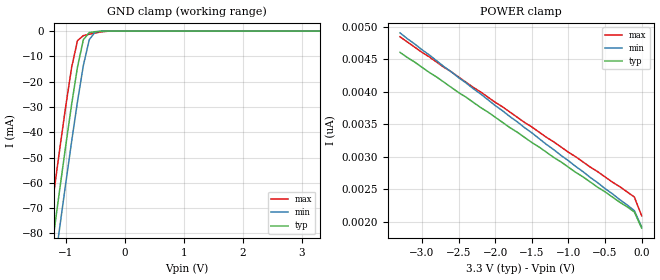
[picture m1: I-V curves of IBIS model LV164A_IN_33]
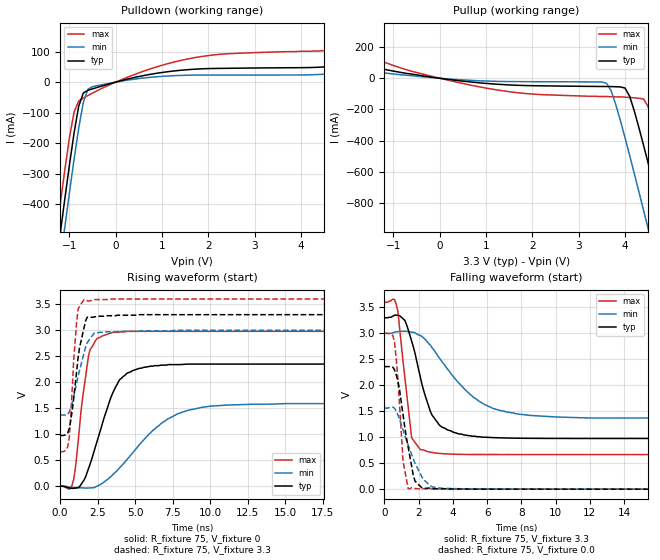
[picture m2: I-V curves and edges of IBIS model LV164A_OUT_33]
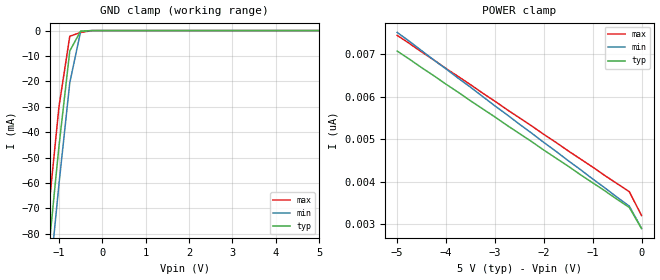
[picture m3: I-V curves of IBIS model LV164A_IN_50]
| TEXAS INSTRUMENTS INCORPORATED
| Standard Linear and Logic Group
| IBIS Model of SN74LV164A
| 8-BIT PARALLEL-OUT SERIAL SHIFT REGISTER
| SOIC 14-pin (D), SOP 14-pin (NS), SSOP 14-pin (DB), TSSOP 14-pin (PW)
| and TVSOP 14-pin (DGV) Package
[IBIS Ver]   3.2
[Comment Char]  |_char
[File Name]   lv164a.ibs
[File Rev]   2.0 H_die
[Date]   May 24, 2000
[Source]   Data created from HSPICE simulations at TI-SLL.
[Notes]   The following is an IBIS list for the LV164A.
|   Please contact sllibis@ti.com with questions and
|   comments concerning SLL IBIS models.
[Disclaimer] Property of Texas Instruments Incorporated.  Unauthorized
   reproduction and/or distribution is strictly prohibited.
   This product is protected under copyright law.
   Created 2000, (C) Copyright 2000, Texas Instruments Inc.,
   All Rights Reserved.
   UNLESS THERE IS A SIGNED, WRITTEN AGREEMENT TO THE
   CONTRARY, TEXAS INSTRUMENTS () IS PROVIDING THE IBIS
   MODELS  AND WITHOUT ANY WARRANTY, EXPRESSED OR
   IMPLIED.  TI assumes no liability for:
   1) the accuracy of the IBIS models provided to your
   company;
   2) the proper functioning of these IBIS Models in your
   design or for any resulting applications; or
   3) infringement of patents, copyrights or intellectual
   property rights resulting from your use of these IBIS
   models.
   TI provides IBIS Models as a service to our customers.
   You and your company shall not distribute, sell or give
   these models to anyone else without prior written
   permission from TI.
   TI reserves the right to make changes to our products or
   to discontinue any semiconductor product or service
   without notice, and advises our customers to obtain the
   latest version of relevant information to verify, before
   placing orders, that the information being relied on is
   current.
   Please be aware that your receipt and use of the IBIS
   information provided shall serve as acceptance of these
   terms and conditions.  If you do not accept these terms,
   you should return or destroy the IBIS models and any
   other accompanying information immediately.
|   Component LV164A_D
[Component]   LV164A_D
[Manufacturer]  Texas Instruments, Inc.
[Package]
|   typ   min   max
R_pkg   0.031   0.028   0.034
L_pkg   3.109nH   2.462nH   3.889nH
C_pkg   0.473pF   0.363pF   0.628pF
[Pin]   signal_name   model_name   R_pin   L_pin   C_pin
1   A   LV164A_IN   0.033   3.854nH   0.622pF
2   B   LV164A_IN   0.032   3.188nH   0.473pF
3   QA   LV164A_OUT   0.028   2.462nH   0.377pF
4   QB   LV164A_OUT   0.031   2.596nH   0.363pF
5   QC   LV164A_OUT   0.028   2.521nH   0.372pF
6   QD   LV164A_OUT   0.034   3.250nH   0.476pF
7   GND   GND   0.034   3.889nH   0.628pF
8   CLK   LV164A_IN   0.034   3.889nH   0.628pF
9   CLR_NOT   LV164A_IN   0.034   3.250nH   0.476pF
10   QE   LV164A_OUT   0.028   2.521nH   0.372pF
11   QF   LV164A_OUT   0.031   2.596nH   0.364pF
12   QG   LV164A_OUT   0.028   2.462nH   0.377pF
13   QH   LV164A_OUT   0.032   3.188nH   0.473pF
14   VCC   POWER   0.033   3.854nH   0.622pF
|   Component LV164A_NS
[Component]   LV164A_NS
[Manufacturer]  Texas Instruments, Inc.
[Package]
|   typ   min   max
R_pkg   0.045   0.039   0.054
L_pkg   3.796nH   2.561nH   4.952nH
C_pkg   0.528pF   0.288pF   0.710pF
[Pin]   signal_name   model_name   R_pin   L_pin   C_pin
1   A   LV164A_IN   0.047   4.867nH   0.706pF
2   B   LV164A_IN   0.051   4.083nH   0.592pF
3   QA   LV164A_OUT   0.041   2.915nH   0.376pF
4   QB   LV164A_OUT   0.039   2.561nH   0.288pF
5   QC   LV164A_OUT   0.041   3.101nH   0.430pF
6   QD   LV164A_OUT   0.047   4.047nH   0.589pF
7   GND   GND   0.051   4.909nH   0.700pF
8   CLK   LV164A_IN   0.045   4.784nH   0.694pF
9   CLR_NOT   LV164A_IN   0.054   4.176nH   0.597pF
10   QE   LV164A_OUT   0.039   3.287nH   0.449pF
11   QF   LV164A_OUT   0.039   2.586nH   0.294pF
12   QG   LV164A_OUT   0.040   2.802nH   0.371pF
13   QH   LV164A_OUT   0.049   4.080nH   0.593pF
14   VCC   POWER   0.052   4.952nH   0.710pF
|   Component LV164A_DB
[Component]   LV164A_DB
[Manufacturer]  Texas Instruments, Inc.
[Package]
|   typ   min   max
R_pkg   0.044   0.041   0.046
L_pkg   3.551nH   3.258nH   3.927nH
C_pkg   0.402pF   0.360pF   0.421pF
[Pin]   signal_name   model_name   R_pin   L_pin   C_pin
1   A   LV164A_IN   0.046   3.927nH   0.408pF
2   B   LV164A_IN   0.044   3.587nH   0.421pF
3   QA   LV164A_OUT   0.041   3.289nH   0.398pF
4   QB   LV164A_OUT   0.042   3.258nH   0.360pF
5   QC   LV164A_OUT   0.041   3.286nH   0.403pF
6   QD   LV164A_OUT   0.044   3.586nH   0.421pF
7   GND   GND   0.046   3.927nH   0.408pF
8   CLK   LV164A_IN   0.046   3.927nH   0.408pF
9   CLR_NOT   LV164A_IN   0.044   3.586nH   0.421pF
10   QE   LV164A_OUT   0.041   3.286nH   0.403pF
11   QF   LV164A_OUT   0.043   3.258nH   0.360pF
12   QG   LV164A_OUT   0.041   3.289nH   0.398pF
13   QH   LV164A_OUT   0.044   3.587nH   0.421pF
14   VCC   POWER   0.046   3.927nH   0.408pF
|   Component LV164A_PW
[Component]   LV164A_PW
[Manufacturer]  Texas Instruments, Inc.
[Package]
|   typ   min   max
R_pkg   0.032   0.029   0.035
L_pkg   2.378nH   2.170nH   2.680nH
C_pkg   0.314pF   0.270pF   0.335pF
[Pin]   signal_name   model_name   R_pin   L_pin   C_pin
1   A   LV164A_IN   0.033   2.618nH   0.330pF
2   B   LV164A_IN   0.031   2.313nH   0.317pF
3   QA   LV164A_OUT   0.030   2.310nH   0.314pF
4   QB   LV164A_OUT   0.031   2.173nH   0.272pF
5   QC   LV164A_OUT   0.030   2.204nH   0.309pF
6   QD   LV164A_OUT   0.032   2.315nH   0.317pF
7   GND   GND   0.035   2.680nH   0.335pF
8   CLK   LV164A_IN   0.033   2.640nH   0.333pF
9   CLR_NOT   LV164A_IN   0.034   2.347nH   0.319pF
10   QE   LV164A_OUT   0.029   2.277nH   0.313pF
11   QF   LV164A_OUT   0.031   2.170nH   0.270pF
12   QG   LV164A_OUT   0.031   2.244nH   0.311pF
13   QH   LV164A_OUT   0.033   2.343nH   0.321pF
14   VCC   POWER   0.035   2.657nH   0.332pF
|   Component LV164A_DGV
[Component]   LV164A_DGV
[Manufacturer]  Texas Instruments, Inc.
[Package]
|   typ   min   max
R_pkg   0.035   0.020   0.045
L_pkg   2.499nH   2.077nH   2.966nH
C_pkg   0.361pF   0.305pF   0.416pF
[Pin]   signal_name   model_name   R_pin   L_pin   C_pin
1   A   LV164A_IN   0.027   2.717nH   0.373pF
2   B   LV164A_IN   0.037   2.434nH   0.398pF
3   QA   LV164A_OUT   0.034   2.200nH   0.316pF
4   QB   LV164A_OUT   0.020   2.077nH   0.309pF
5   QC   LV164A_OUT   0.030   2.147nH   0.305pF
6   QD   LV164A_OUT   0.042   2.580nH   0.408pF
7   GND   GND   0.039   2.921nH   0.385pF
8   CLK   LV164A_IN   0.033   2.841nH   0.380pF
9   CLR_NOT   LV164A_IN   0.042   2.611nH   0.410pF
10   QE   LV164A_OUT   0.038   2.331nH   0.329pF
11   QF   LV164A_OUT   0.026   2.223nH   0.319pF
12   QG   LV164A_OUT   0.034   2.259nH   0.313pF
13   QH   LV164A_OUT   0.045   2.681nH   0.416pF
14   VCC   POWER   0.042   2.966nH   0.386pF
[Model Selector]   LV164A_IN
LV164A_IN_33   3.3-V Vcc Input Model
LV164A_IN_50   5.0-V Vcc Input Model
[Model Selector]   LV164A_OUT
LV164A_OUT_33   3.3-V Vcc Output Model
LV164A_OUT_50   5.0-V Vcc Output Model
| Models and submodels in the file (4): LV164A_IN_33 (Input), LV164A_OUT_33 (Output), LV164A_IN_50 (Input), LV164A_OUT_50 (Output)
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|   Model LV164A_IN_33
[Model]   LV164A_IN_33
Model_type  Input
Polarity   Inverting
Vinl = 0.99
Vinh = 2.31
| variable   typ   min   max
C_comp   1.24pf   0.94pf   1.54pf
[Temperature Range]   25   85   -40
[Voltage Range]   3.3   3.0   3.6
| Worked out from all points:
|   GND clamp passes 1 mA (typ) near -0.61 V on its own axis
[GND Clamp]
|   Voltage   I(typ)   I(min)   I(max)
-3.3V     -460mA     -475mA     -445mA
-1.3V     -97.5mA    -113mA     -81.5mA
-1.2V     -79.9mA    -95mA      -63.9mA
-1.1V     -62.6mA    -77.6mA    -46.7mA
-1V       -45.6mA    -60.5mA    -30mA
-900mV    -29.2mA    -43.9mA    -14.6mA
-800mV    -14.3mA    -28mA      -3.81mA
-700mV    -3.42mA    -13.6mA    -1.78mA
-600mV    -581uA     -3.4mA     -1.25mA
-500mV    -233uA     -353uA     -759uA
-400mV    -58.1uA    -21.9uA    -324uA
3.3V      1.9nA      2.34nA     1.69nA
[POWER Clamp]
|   Voltage   I(typ)   I(min)   I(max)
-3.3V     4.61nA     4.91nA     4.85nA
-3V       4.38nA     4.65nA     4.61nA
-100mV    2.15nA     2.17nA     2.38nA
0V        1.9nA      1.92nA     2.09nA
|   Model LV164A_OUT_33
[Model]   LV164A_OUT_33
Model_type  Output
Polarity   Non-Inverting
Vmeas = 1.65v
Cref = 15pf
| variable   typ   min   max
C_comp   4.62pf   3.47pf   5.77pf
[Temperature Range]   25   85   -40
[Voltage Range]   3.3   3.0   3.6
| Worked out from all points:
|   slope of the pulldown table from 0 to 0.495 V, typ, clamps not added: 27.3 ohm
|   slope of the pullup table from 0 to 0.495 V, typ, clamps not added: 27.2 ohm
|   rising waveform, R_fixture 75, V_fixture 0: 20-80 % time 1.6ns typ, 3.21ns min, 723ps max; typ from 0 V to 2.35 V
|   falling waveform, R_fixture 75, V_fixture 3.3: 20-80 % time 1.16ns typ, 2.61ns min, 585ps max; typ from 3.3 V to 0.976 V
|   rising waveform, R_fixture 75, V_fixture 3.3: 20-80 % time 632ps typ, 815ps min, 375ps max; typ from 0.976 V to 3.3 V
|   falling waveform, R_fixture 75, V_fixture 0.0: 20-80 % time 677ps typ, 1.09ns min, 359ps max; typ from 2.36 V to 0 V
[Pulldown]
|   Voltage   I(typ)   I(min)   I(max)
-3.3V     -3.04A     -3.13A     -2.95A
-1.3V     -615mA     -707mA     -518mA
-1.2V     -498mA     -591mA     -401mA
-1.1V     -383mA     -475mA     -288mA
-900mV    -167mA     -253mA     -98.6mA
-800mV    -79.1mA    -151mA     -61.7mA
-700mV    -35.5mA    -66.4mA    -51.9mA
-600mV    -26.8mA    -23.2mA    -43.9mA
-500mV    -22mA      -14.7mA    -35.8mA
1.6V      41.2mA     22.8mA     77.1mA
4.7V      52.3mA     27.8mA     106mA
6.6V      95.5mA     55.2mA     176mA
[Pullup]
|   Voltage   I(typ)   I(min)   I(max)
-3.3V     172mA      95.9mA     319mA
500mV     -18.4mA    -10.6mA    -33.4mA
3.6V      -52.9mA    -31.5mA    -117mA
3.8V      -54.2mA    -168mA     -119mA
4V        -62.6mA    -381mA     -121mA
4.1V      -115mA     -494mA     -123mA
4.4V      -429mA     -845mA     -133mA
4.5V      -544mA     -964mA     -182mA
4.8V      -899mA     -1.32A     -505mA
4.9V      -1.02A     -1.44A     -622mA
5.2V      -1.38A     -1.81A     -981mA
6.6V      -3.09A     -3.52A     -2.69A
[Ramp]
| variable   typ   min   max
dV/dt_r   1.42E+00/1.59E-09   9.66E-01/3.30E-09   1.79E+00/6.80E-10
dV/dt_f   1.43E+00/1.14E-09   1.00E+00/2.67E-09   1.80E+00/5.30E-10
R_load = 75
[Rising Waveform]
R_fixture = 75
V_fixture = 0
|   Time   V(typ)   V(min)   V(max)
0s        0V         0V         0V
900ps     -38.3mV    -22.6mV    130mV
1.5ns     81.2mV     -30mV      1.71V
1.9ns     348mV      -31.9mV    2.52V
2.8ns     1.19V      55.5mV     2.89V
3.5ns     1.79V      221mV      2.96V
4.4ns     2.16V      495mV      2.98V
6.4ns     2.32V      1.13V      2.98V
8.5ns     2.35V      1.46V      2.98V
25ns      2.35V      1.59V      2.98V
[Falling Waveform]
R_fixture = 75
V_fixture = 3.3
V_fixture_min = 3.0
V_fixture_max = 3.6
|   Time   V(typ)   V(min)   V(max)
0s        3.3V       3V         3.6V
700ps     3.35V      3.03V      3.56V
1.2ns     3.25V      3.04V      2.16V
1.6ns     2.85V      3.02V      989mV
2.1ns     2.17V      2.96V      762mV
2.7ns     1.49V      2.77V      712mV
3.3ns     1.21V      2.49V      685mV
5.2ns     1.02V      1.77V      668mV
7.2ns     984mV      1.48V      666mV
25ns      976mV      1.37V      666mV
[Rising Waveform]
R_fixture = 75
V_fixture = 3.3
V_fixture_min = 3.0
V_fixture_max = 3.6
|   Time   V(typ)   V(min)   V(max)
0s        976mV      1.37V      666mV
400ps     991mV      1.37V      699mV
600ps     1.11V      1.43V      919mV
900ps     1.68V      1.72V      2.41V
1.1ns     2.21V      1.99V      3.17V
1.2ns     2.48V      2.12V      3.41V
1.6ns     3.06V      2.57V      3.59V
2.2ns     3.25V      2.92V      3.58V
2.9ns     3.27V      2.97V      3.59V
25ns      3.3V       3V         3.6V
[Falling Waveform]
R_fixture = 75
V_fixture = 0.0
|   Time   V(typ)   V(min)   V(max)
0s        2.36V      1.56V      3V
400ps     2.36V      1.58V      2.99V
600ps     2.3V       1.56V      2.83V
800ps     2.08V      1.43V      2.11V
1.1ns     1.43V      1.14V      529mV
1.4ns     800mV      847mV      9.99mV
1.8ns     153mV      497mV      12.5mV
2.3ns     11.5mV     184mV      9.19mV
3.2ns     6.92mV     23.2mV     3.05mV
25ns      0V         0V         6.22uV
|   Model LV164A_IN_50
[Model]   LV164A_IN_50
Model_type  Input
Polarity   Inverting
Vinl = 1.5
Vinh = 3.5
| variable   typ   min   max
C_comp   1.24pf   0.94pf   1.54pf
[Temperature Range]   25   85   -40
[Voltage Range]   5.0   4.5   5.5
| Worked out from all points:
|   GND clamp passes 1 mA (typ) near -0.52 V on its own axis
[GND Clamp]
|   Voltage   I(typ)   I(min)   I(max)
-5V       -773mA     -786mA     -758mA
-1.5V     -133mA     -148mA     -117mA
-1.25V    -88.7mA    -104mA     -72.7mA
-1V       -45.6mA    -60.5mA    -30mA
-750mV    -7.99mA    -20.5mA    -2.23mA
-500mV    -233uA     -353uA     -759uA
-250mV    -2.63nA    -182nA     -26.9uA
5V        2.9nA      3.64nA     2.54nA
[POWER Clamp]
|   Voltage   I(typ)   I(min)   I(max)
-5V       7.08nA     7.52nA     7.45nA
-1.5V     4.37nA     4.5nA      4.73nA
-250mV    3.4nA      3.43nA     3.77nA
0V        2.9nA      2.91nA     3.21nA
